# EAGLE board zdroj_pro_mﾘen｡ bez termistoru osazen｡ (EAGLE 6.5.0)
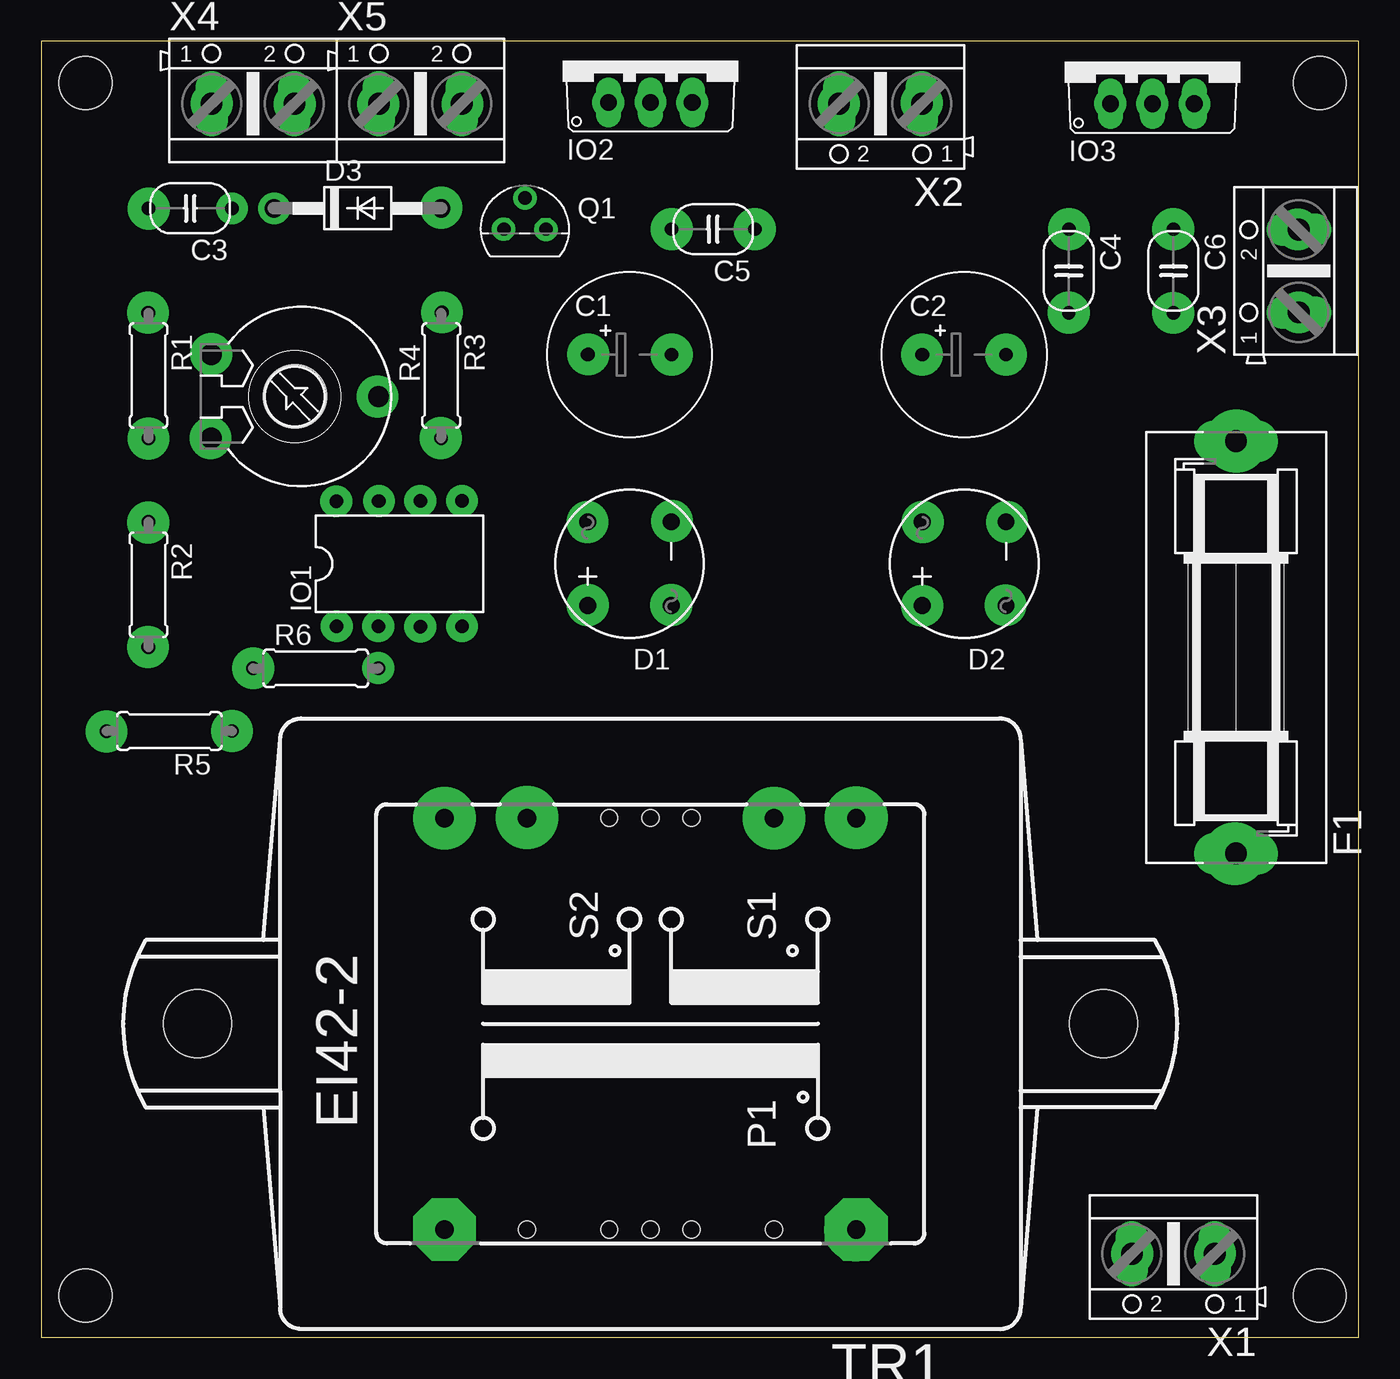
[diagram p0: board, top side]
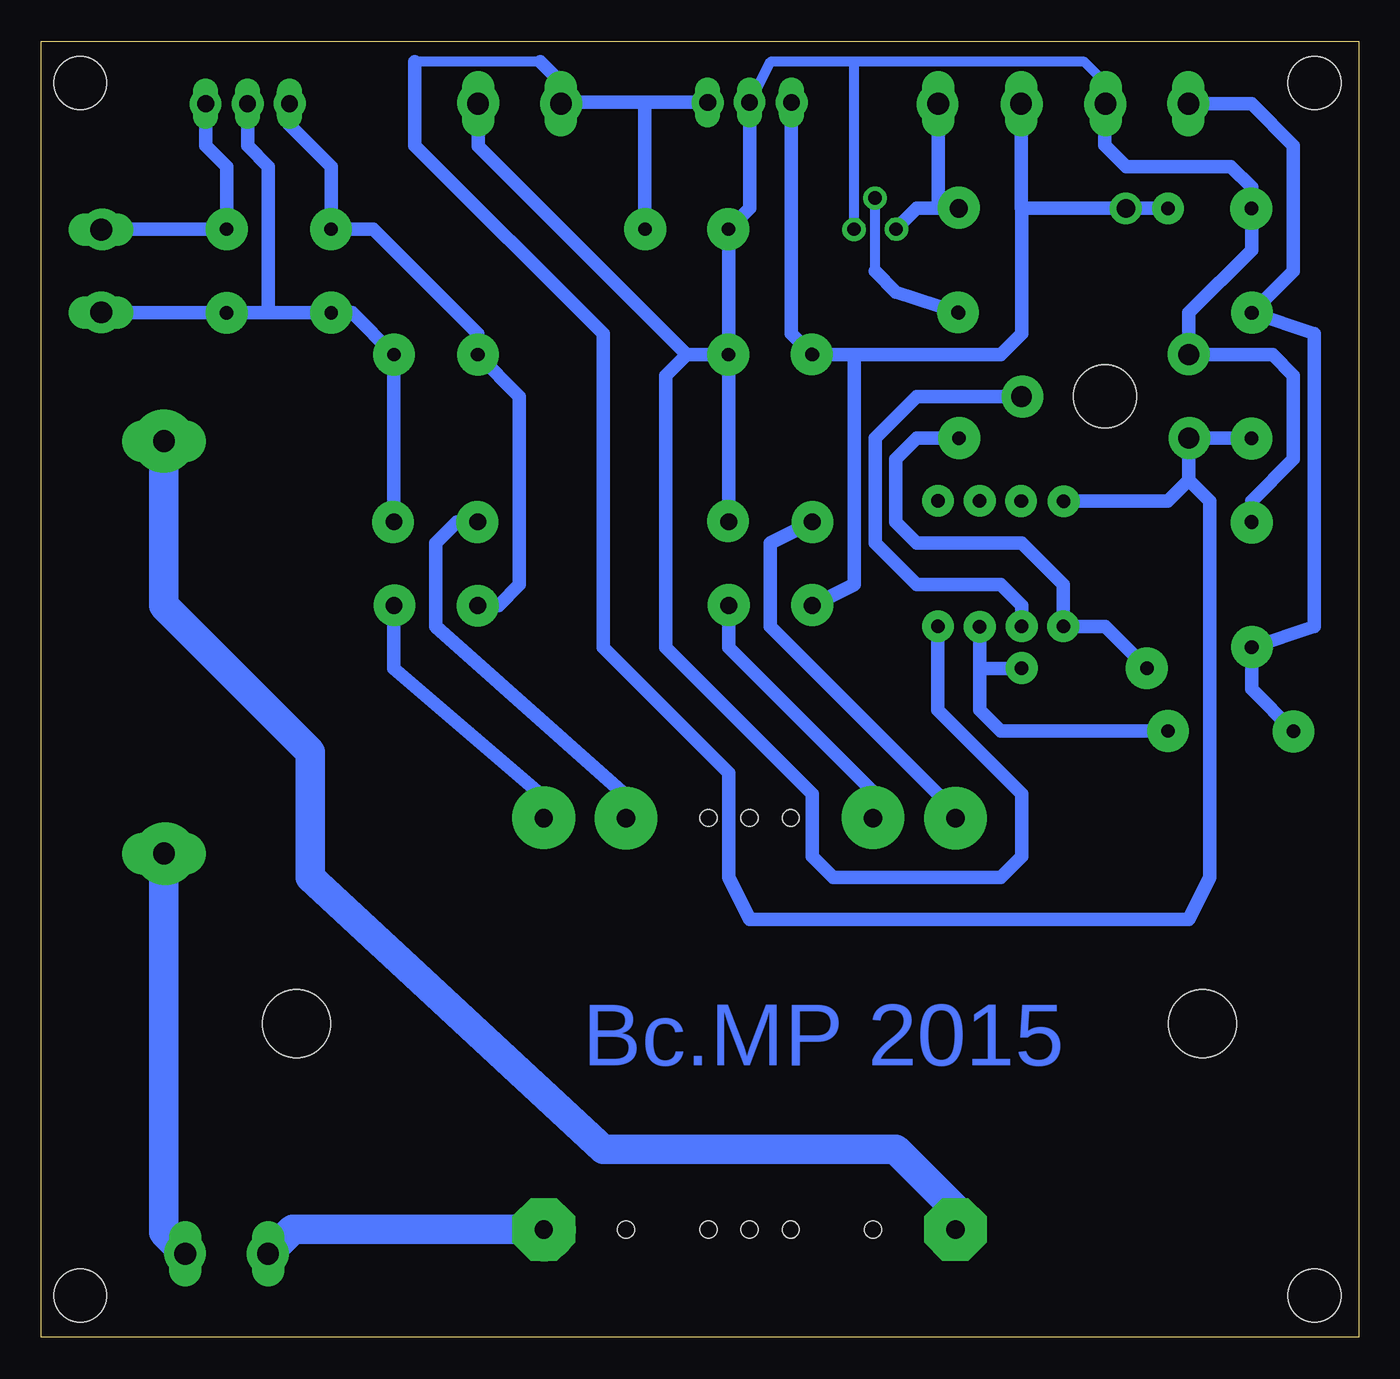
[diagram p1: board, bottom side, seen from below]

Size 80 x 78.73 mm. Coordinates in mm from the lower left corner, seen from the top.
Outline: 0,0 80,0 80,78.73 0,78.73 0,0
Copper layers (1*16): Top 0.035mm / dielectric 1.5mm / Bottom 0.035mm
Design rules "default": minimum track width 10mil, minimum drill 24mil, track to track 8mil, track to pad 8mil, pad to pad 8mil, via to via 8mil, smd to smd 8mil, copper to edge 40mil, drill to drill 8mil, minimum pad ring 10mil, minimum via ring 8mil, stop-mask expansion 4mil, vias tented up to drill 0mil, thermal gap 10mil
Holes 3.2 mm at 2.7,76.2 77.63,76.2 77.63,2.54 2.7,2.54

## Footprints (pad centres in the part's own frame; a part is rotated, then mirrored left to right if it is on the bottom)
E5-10 = drill 0.813 pad 1.778: + -2.54,0 | drill 0.813 pad 1.778 octagon: - 2.54,0
C3X5 = drill 0.813 pad 1.422 octagon: 1 -2.54,0; 2 2.54,0
WOM = drill 1.016 pad 1.676: + -2.54,2.54 | drill 1.016 pad 1.676 octagon: - 2.54,-2.54; AC1 2.54,2.54; AC2 -2.54,-2.54
DO41-10 = drill 1.118 pad 1.778 octagon: A 5.08,0 | drill 1.118 pad 1.778: C -5.08,0
SH25 = drill 1.321 pad 2.54 long: 1 -12.522,0; 2 12.522,0
DIL08 = drill 0.813 pad 1.27: 1 -3.81,-3.81; 2 -1.27,-3.81; 3 1.27,-3.81; 4 3.81,-3.81; 5 3.81,3.81; 6 1.27,3.81; 7 -1.27,3.81; 8 -3.81,3.81
TO220V = drill 1.016 long: 1 -2.54,-2.54; 2 0,-2.54; 3 2.54,-2.54
TO92 = drill 0.813 octagon: 1 1.27,0; 2 0,1.905; 3 -1.27,0
0207/7 = drill 0.813 octagon: 1 -3.81,0; 2 3.81,0
PT10V = drill 1.27 octagon: A -2.54,-5.08; E 2.54,-5.08; S 0,5.08 | hole 3.81: 0,0
TO92' = drill 0.813 pad 1.422 octagon: 1 -1.27,0; 2 1.27,0
EI42-2B = drill 1.118 pad 3.81 octagon: 1 -12.497,12.497; 5 -12.497,-12.497 | drill 1.118 pad 3.175 octagon: 6 12.497,-12.497; 7 12.497,-7.493; 9 12.497,7.493; 10 12.497,12.497 | hole 4.115: 0,-27.508; 0,27.508 | hole 1.016: -12.5,7.5; -12.5,0; -12.5,-7.5; 12.5,0; -12.5,2.5; -12.5,-2.5; 12.5,2.5; 12.5,-2.5
AK500/2 = drill 1.321 long: 1 -2.515,0; 2 2.515,0

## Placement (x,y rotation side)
C1  [E5-10]  35.72,59.69 0 top
C2  [E5-10]  56.04,59.69 0 top
C3  [C3X5]  9.05,68.58 180 top
C4  [C3X5]  62.39,64.77 270 top
C5  [C3X5]  40.8,67.31 180 top
C6  [C3X5]  68.74,64.77 270 top
D1  B250C1500  [WOM]  35.72,46.99 90 top
D2  B250C1500  [WOM]  56.04,46.99 90 top
D3  1N4007  [DO41-10]  19.21,68.58 0 top
F1  [SH25]  72.55,41.91 90 top
IO1  LM358N  [DIL08]  21.75,46.99 0 top
IO2  7809  [TO220V]  36.99,77.55 0 top
IO3  7809  [TO220V]  67.47,77.47 0 top
Q1  BC337  [TO92]  29.37,67.31 0 top
R1  [0207/7]  6.51,58.42 270 top
R2  [0207/7]  6.51,45.72 270 top
R3  [0207/7]  24.29,58.42 270 top
R4  [PT10V]  15.4,57.15 270 top
R5  [0207/7]  7.78,36.83 180 top
R6  [0207/7]  16.67,40.64 0 top
RT1  [TO92']  not placed on the board
TR1  [EI42-2B]  36.99,19.05 90 top
X1  [AK500/2]  68.74,5.08 180 top
X2  [AK500/2]  50.96,74.93 180 top
X3  [AK500/2]  76.36,64.77 90 top
X4  [AK500/2]  12.86,74.93 0 top
X5  [AK500/2]  23.02,74.93 0 top

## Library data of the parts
C1 C2 = elektrolyticke kondenzatory radialni
C3-C6 = kondenzatory
D1 D2 = diodove mustky a diaky
D3 = diody
F1 = pojistky; MF: SCHURTER; MPN: 0031.8211; OC_FARNELL: 1162741; OC_NEWARK: 96B9380
IO1 = IO linear
IO2 IO3 = linear
Q1 = tranzistory NPN
R1-R3 R5 R6 = rezistory
R4 = odporove trimry
RT1 = termistory
TR1 = transformatory
X1-X5 = Konektory; OC_FARNELL: unknown; OC_NEWARK: unknown

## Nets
N$1: F1.1 X1.1
N$2: F1.2 TR1.1
N$3: D1.AC1 TR1.10
N$4: D1.AC2 TR1.9
N$5: D2.AC1 TR1.7
N$6: D2.AC2 TR1.6
N$7: C1.+ C3.1 D1.+ D3.C IO2.1 X5.1
N$10: C2.+ C4.1 D2.+ IO3.1
N$11: C6.1 IO3.3 X3.2
N$13: TR1.5 X1.2
N$14: D3.A Q1.3 X5.2
N$15: R1.1 R2.2 R5.2 X4.1
N$16: IO1.2 R4.S
N$17: Q1.2 R3.1
N$18: IO1.1 R3.2 R6.1
N$19: IO1.3 R5.1 R6.2
N$20: C2.- C4.2 C6.2 D2.- IO3.2 X3.1
V+: C5.1 IO1.8 IO2.3 R1.2 R4.E X2.2
V-: C1.- C3.2 C5.2 D1.- IO1.4 IO2.2 Q1.1 R2.1 R4.A X2.1 X4.2

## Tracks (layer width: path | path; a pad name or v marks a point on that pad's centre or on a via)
N$1
  Bottom 1.778: F1.1 72.55,6.38 X1.1
N$2
  Bottom 0.813: TR1.1 24.49,7.82 | 72.55,54.61 F1.2
  Bottom 1.778: 24.49,7.82 28.1,11.43 45.88,11.43 63.66,27.94 63.66,35.56 72.55,44.45 72.55,54.61
N$3
  Bottom 0.813: D1.AC1 35.72,48.26 35.72,43.18 24.49,31.95 TR1.10
N$4
  Bottom 0.813: TR1.9 29.5,33.15 38.26,41.91 D1.AC2
N$5
  Bottom 0.813: TR1.7 44.48,32.89 56.04,43.18 56.04,48.26 54.77,49.53 D2.AC1
N$6
  Bottom 0.813: TR1.6 49.49,32.82 58.58,40.64 D2.AC2
N$7
  Bottom 0.813: D1.+ 30.64,45.72 30.64,59.69 | X5.1 20.5,69.83 20.5,68.58 | IO2.1 34.45,60.96 C1.+ 30.64,59.69 | 20.5,68.58 19.23,68.58 D3.C C3.1 | 30.64,59.69 21.75,59.69 20.48,60.96 20.48,68.56 20.5,68.58
N$8  (via drill 0.8 pad 2.54)
  other vias: 3.96,36.79
N$9  (via drill 0.8 pad 2.54)
  other vias: 11.58,36.83
N$10
  Bottom 0.406: D2.+ 52.23,44.45
  Bottom 0.813: 52.23,44.45 50.96,45.72 50.96,57.15 C2.+ 53.5,60.96 59.85,67.31 C4.1 62.39,71.12 64.93,73.66 IO3.1
N$11
  Bottom 0.406: 76.33,67.31 X3.2
  Bottom 0.813: 76.33,67.31 C6.1 68.74,71.12 70.01,72.39 IO3.3
N$12  (via drill 0.8 pad 2.54)
  other vias: 12.87,40.65
N$13
  Bottom 1.778: TR1.5 64.73,6.55 66.2,5.08 X1.2
N$14
  Bottom 0.813: D3.A 25.56,68.58 | 25.56,68.58 26.83,68.58 Q1.3 | X5.2 25.53,68.61 25.56,68.58
N$15
  Bottom 0.813: X4.1 6.51,74.93 3.97,72.39 3.97,64.77 R1.1 2.7,60.96 2.7,43.18 R2.2 6.51,39.37 R5.2
N$16
  Bottom 0.813: IO1.2 20.48,44.45 21.75,45.72 26.83,45.72 29.37,48.26 29.37,54.61 26.83,57.15 R4.S
N$17
  Bottom 0.61: 29.37,64.77 Q1.2
  Bottom 0.813: R3.1 28.1,63.5 29.37,64.77
N$18
  Bottom 0.813: R3.2 26.83,54.61 28.1,53.34 28.1,49.53 26.83,48.26 20.48,48.26 17.94,45.72 IO1.1 15.4,43.18 R6.1
N$19
  Bottom 0.813: IO1.3 23.02,40.64 | 23.02,40.64 23.02,38.1 21.75,36.83 R5.1 | R6.2 23.02,40.64
N$20
  Bottom 0.406: 76.33,62.23 X3.1
  Bottom 0.813: D2.- C2.- 61.12,62.23 C4.2 66.2,62.23 | 66.2,62.23 C6.2 76.33,62.23 | IO3.2 67.47,72.39 66.2,71.12 66.2,62.23
N$21  (via drill 0.8 pad 2.54)
  other vias: 6.49,41.93
N$22  (via drill 0.8 pad 1.93)
  other vias: 17.95,43.19
N$23  (via drill 0.8 pad 1.93)
  other vias: 20.47,43.19
N$24  (via drill 0.8 pad 1.93)
  other vias: 23.02,43.16
N$25  (via drill 0.8 pad 1.93)
  other vias: 25.56,43.19
N$26  (via drill 0.8 pad 1.93)
  other vias: 25.55,50.82
N$27  (via drill 0.8 pad 1.93)
  other vias: 23.02,50.82
N$28  (via drill 0.8 pad 1.93)
  other vias: 20.51,50.8
N$29  (via drill 0.8 pad 1.93)
  other vias: 17.92,50.78
N$30  (via drill 0.6 pad 1.42)
  other vias: 28.07,67.31
N$31  (via drill 0.6 pad 1.42)
  other vias: 30.65,67.28
N$32  (via drill 0.6 pad 1.42)
  other vias: 29.39,69.19
N$33  (via drill 0.8 pad 2.54)
  other vias: 33.17,49.53
N$34  (via drill 0.8 pad 2.54)
  other vias: 38.3,49.57
N$35  (via drill 0.8 pad 2.54)
  other vias: 38.26,44.48
N$36  (via drill 0.8 pad 2.54)
  other vias: 33.19,44.48
N$37  (via drill 0.8 pad 2.54)
  other vias: 24.26,54.63
N$38  (via drill 0.8 pad 2.54)
  other vias: 24.34,62.26
N$39  (via drill 0.8 pad 2.54)
  other vias: 20.42,57.14
N$40  (via drill 0.8 pad 2.54)
  other vias: 10.32,59.73
N$41  (via drill 0.8 pad 2.54)
  other vias: 10.29,54.63
N$42  (via drill 0.8 pad 2.54)
  other vias: 6.51,49.49
N$43  (via drill 0.8 pad 2.54)
  other vias: 6.51,54.6
N$44  (via drill 0.8 pad 2.54)
  other vias: 6.49,62.23
N$45  (via drill 0.8 pad 2.54)
  other vias: 33.21,59.7
N$46  (via drill 0.8 pad 2.54)
  other vias: 38.28,59.68
N$47  (via drill 0.8 pad 2.54)
  other vias: 6.53,68.55
N$48  (via drill 0.8 pad 1.93)
  other vias: 14.15,68.57
N$49  (via drill 0.8 pad 1.93)
  other vias: 11.58,68.57
N$50  (via drill 0.8 pad 2.54)
  other vias: 24.28,68.61
N$51  (via drill 0.8 pad 2.54)
  other vias: 38.28,67.31
N$52  (via drill 0.8 pad 2.54)
  other vias: 43.32,67.31
N$53  (via drill 0.8 pad 2.54)
  other vias: 62.4,67.31
N$54  (via drill 0.8 pad 2.54)
  other vias: 68.73,67.31
N$55  (via drill 0.8 pad 2.54)
  other vias: 68.73,62.23
N$56  (via drill 0.8 pad 2.54)
  other vias: 62.39,62.24
N$57  (via drill 0.8 pad 2.54)
  other vias: 53.48,59.68
N$58  (via drill 0.8 pad 2.54)
  other vias: 58.58,59.68
N$59  (via drill 0.8 pad 2.54)
  other vias: 53.53,49.52
N$60  (via drill 0.8 pad 2.54)
  other vias: 58.64,49.52
N$61  (via drill 0.8 pad 2.54)
  other vias: 58.55,44.47
N$62  (via drill 0.8 pad 2.54)
  other vias: 53.5,44.44
N$63  (via drill 0.8 pad 3.81)
  other vias: 24.49,6.55
N$64  (via drill 0.8 pad 3.81)
  other vias: 49.45,6.53
N$65  (via drill 0.8 pad 3.81)
  other vias: 44.5,31.54
N$66  (via drill 0.8 pad 3.81)
  other vias: 49.48,31.56
N$67  (via drill 0.8 pad 3.81)
  other vias: 29.5,31.59
N$68  (via drill 0.8 pad 3.81)
  other vias: 24.49,31.54
N$69  (via drill 0.8 pad 3.81)
  other vias: 72.47,29.38
N$70  (via drill 0.8 pad 3.81)
  other vias: 72.56,54.44
N$71  (via drill 0.8 pad 1.93)
  other vias: 70.03,74.92
N$72  (via drill 0.8 pad 1.93)
  other vias: 67.46,74.92
N$73  (via drill 0.8 pad 1.93)
  other vias: 64.91,74.95
N$74  (via drill 0.8 pad 1.93)
  other vias: 34.43,75.01
N$75  (via drill 0.8 pad 1.93)
  other vias: 37,75.03
N$76  (via drill 0.8 pad 1.93)
  other vias: 39.53,74.99
N$77  (via drill 0.8 pad 2.54)
  other vias: 76.34,62.26
N$78  (via drill 0.8 pad 2.54)
  other vias: 76.3,67.29
N$79  (via drill 0.8 pad 2.54)
  other vias: 25.58,74.91
N$80  (via drill 0.8 pad 2.54)
  other vias: 20.47,74.91
N$81  (via drill 0.8 pad 2.54)
  other vias: 15.39,74.91
N$82  (via drill 0.8 pad 2.54)
  other vias: 10.35,74.95
N$83  (via drill 0.8 pad 2.54)
  other vias: 48.43,74.92
N$84  (via drill 0.8 pad 2.54)
  other vias: 53.46,74.99
N$85  (via drill 0.8 pad 2.54)
  other vias: 71.26,5.1
N$86  (via drill 0.8 pad 2.54)
  other vias: 66.23,5.08
N$87  (via drill 0.8 pad 1.93)
  other vias: 20.47,40.67
V+
  Bottom 0.61: 48.42,74.93 48.42,76.2 | 49.69,77.47 57.31,77.47
  Bottom 0.813: R1.2 R4.E 10.32,52.07 | IO2.3 43.34,75.01 | 43.34,75.01 48.37,75.01 X2.2 48.42,74.93 | C5.1 43.34,75.01 | 10.32,52.07 9.05,50.8 9.05,27.94 10.32,25.4 36.99,25.4 38.26,27.94 38.26,34.29 45.88,41.91 45.88,60.96 57.31,72.39 57.31,77.47 | IO1.8 11.59,50.8 10.32,52.07 | 48.42,76.2 49.69,77.47
V-
  Bottom 0.61: Q1.1 30.64,77.47 | 30.64,77.47 35.72,77.47 IO2.2 | X4.2 15.38,76.17 16.67,77.47 30.64,77.47
  Bottom 0.813: IO1.4 25.56,38.1 20.48,33.02 20.48,29.21 21.75,27.94 31.91,27.94 33.18,29.21 33.18,33.02 42.07,41.91 42.07,58.42 40.8,59.69 | D1.- C1.- | X4.2 15.43,72.42 14.13,71.12 7.78,71.12 6.51,69.85 C3.2 6.51,66.04 10.32,62.23 R4.A 5.24,59.69 3.97,58.42 3.97,53.34 6.51,50.8 R2.1 | IO2.2 36.99,68.58 C5.2 C1.- | X2.1 53.48,72.36 40.8,59.69 | 40.8,59.69 C1.-

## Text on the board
Bottom: Bc.MP 2015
